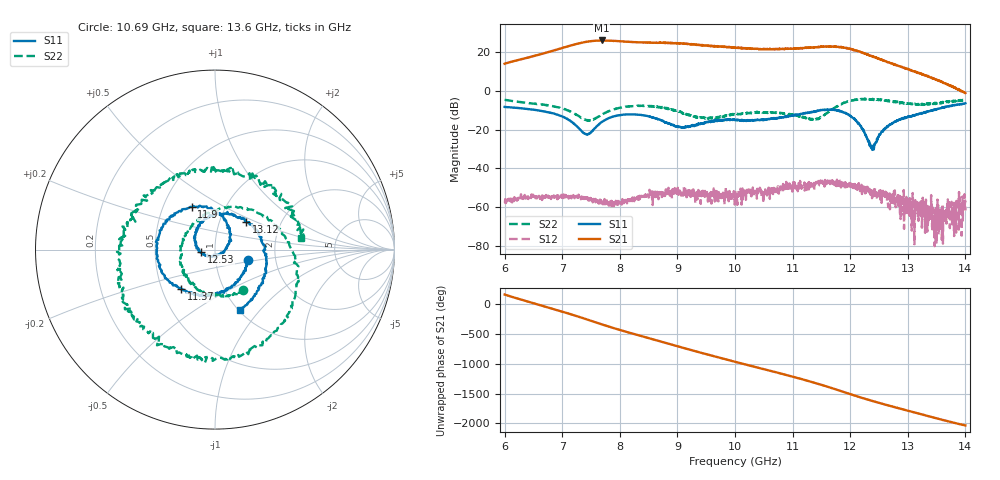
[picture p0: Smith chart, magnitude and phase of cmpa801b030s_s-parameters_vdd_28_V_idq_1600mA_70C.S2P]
!Keysight Technologies,E5071C,MY46110325,B.14.03
!Date: Fri Aug 07 15:36:05 2020
!Data & Calibration Information:
!Freq	S11:SOLT2(ON)	S21:SOLT2(ON)	S12:SOLT2(ON)	S22:SOLT2(ON)
!PortZ  Port1:50+j0  Port2:50+j0
!Above PortZ is port z conversion or system Z0 setting when saving the data.
!When reading, reference impedance value at option line is always used.
# Hz S dB R 50
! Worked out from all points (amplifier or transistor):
!   1601 points, 6 GHz to 14 GHz, reference 50 ohm
!   highest |S21| = 26.0 dB at 7.685 GHz (marker M1)
!   |S21| within 3 dB of that: 7.103 GHz to 9.573 GHz (2.47 GHz wide, 29.6 % of centre)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
!   unconditionally stable (mu >= 1): start of sweep to end of sweep
!   at 7.33 GHz: K = 16.96, MAG = 25.0 dB, |S12| = -55.8 dB
!   at 10 GHz: K = 22.07, MAG = 22.7 dB, |S12| = -56.0 dB
!   at 14 GHz: K = 349.80, MAG = 1.9 dB, |S12| = -61.8 dB
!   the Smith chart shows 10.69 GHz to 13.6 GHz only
!   S11 on the Smith chart (normalised r, x): 10.69 GHz: 1.44, -0.17; 11.37 GHz: 0.63, -0.30; 11.9 GHz: 0.70, +0.36; 12.53 GHz: 0.85, -0.02; 13.12 GHz: 1.34, +0.44; 13.6 GHz: 1.01, -0.79
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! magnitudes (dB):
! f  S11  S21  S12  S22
! 6 GHz  -8.3  14.0  -58.0  -4.6
! 6.865 GHz  -11.8  20.9  -54.4  -8.1
! 7.335 GHz  -20.8  24.9  -55.5  -14.0
! 7.46 GHz  -22.2  25.5  -55.6  -15.2
! 7.685 GHz  -16.2  26.0  -57.1  -12.4
! 8.13 GHz  -12.2  25.4  -56.3  -8.2
! 8.67 GHz  -14.8  24.9  -56.0  -8.3
! 9.09 GHz  -19.1  24.3  -54.0  -11.4
! 10 GHz  -15.0  22.3  -56.0  -12.1
! 10.69 GHz  -14.3  21.5  -50.3  -11.2
! 11.34 GHz  -11.0  22.4  -49.0  -14.7
! 11.37 GHz  -10.7  22.5  -47.6  -14.8
! 11.9 GHz  -11.4  22.3  -47.4  -6.1
! 12.15 GHz  -16.7  20.5  -47.7  -4.3
! 12.38 GHz  -29.6  17.9  -52.7  -4.5
! 12.53 GHz  -22.0  16.2  -56.4  -5.0
! 12.67 GHz  -17.8  14.7  -54.6  -5.0
! 13.12 GHz  -12.7  9.9  -65.0  -6.8
! 13.39 GHz  -10.3  6.9  -64.9  -6.7
! 13.46 GHz  -9.8  6.2  -63.8  -6.4
! 13.6 GHz  -8.8  4.5  -60.5  -6.3
! 14 GHz  -6.4  -1.1  -61.8  -4.5
